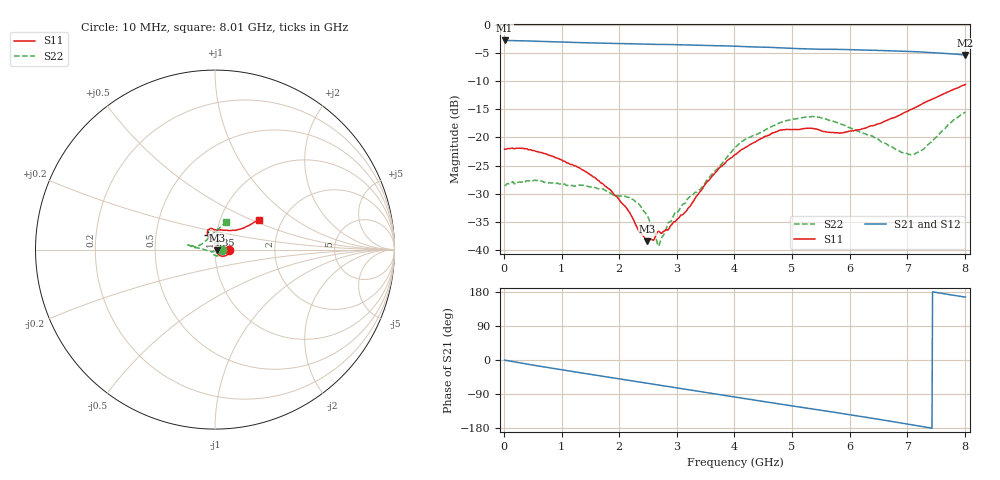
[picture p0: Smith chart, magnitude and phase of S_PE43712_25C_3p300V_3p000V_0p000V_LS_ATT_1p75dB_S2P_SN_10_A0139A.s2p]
! DEVICE ID: PE43712
! File Path: z:\PE43713\PE43713_CHAR_NOM_04292014\AMB\3p300\LS_ATT_1p75dB\PE43713_AMB_3p300V_3p000V_0p000V_LS_ATT_1p75dB_S2P_SN_10_A0139A.s2p
! Serial: 10
! Lot: A0139A
! Temp: 25C
! VDD: 3.300
! VSS: 0.000
! Control_Hi: 3.000
! Control_Lo: 0.000
! Attenuation Step: 1.75dB
! Port 1: RF1
! Port 2: RF2
! ThroughPath:1-2
! IDD: 0.0001468347
! ISS: -9.22e-008
#  Hz  S  RI  R  50
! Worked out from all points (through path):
!   801 points, 10 MHz to 8.01 GHz, reference 50 ohm
!   highest |S21| = -2.79 dB at 10 MHz (marker M1); lowest = -5.4 dB at 8.01 GHz (marker M2)
!   group delay of S21, straight-line fit = 66.5 ps
!   lowest |S11| = -38.4 dB at 2.49 GHz (marker M3), VSWR 1.02, Z = 51.2 - j0.349 ohm
!   |S11| at or under -10 dB: start of sweep to end of sweep
!   |S22| runs from -39.3 to -15.5 dB; largest |S21 - S12| = 0.0022
!   S11 on the Smith chart (normalised r, x): 10 MHz: 1.17, -0.00; 4.35 GHz: 0.91, +0.15; 8.01 GHz: 1.52, +0.55
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1e7  0.0788 -0.000465  0.7254 -0.00398  0.7253 -0.00389  0.0376 -0.000487
6.3e8  0.0679 -0.0283  0.6822 -0.204  0.6818 -0.204  0.0342 -0.0225
1.35e9  0.0364 -0.0369  0.5734 -0.3904  0.5732 -0.3903  0.013 -0.0352
1.84e9  0.0208 -0.0276  0.4764 -0.491  0.4763 -0.4908  0.00131 -0.0322
2.2e9  0.0121 -0.0167  0.3943 -0.5521  0.3944 -0.5518  -0.00773 -0.028
2.35e9  0.0109 -0.00944  0.3574 -0.5733  0.3575 -0.5732  -0.00783 -0.0241
2.49e9  0.0115 -0.00341  0.322 -0.5905  0.3221 -0.5905  -0.00889 -0.018
2.58e9  0.0122 0.00198  0.2991 -0.5996  0.2994 -0.5998  -0.00917 -0.0131
2.68e9  0.0128 0.00724  0.2748 -0.6099  0.275 -0.6098  -0.00668 -0.00853
2.83e9  0.00986 0.0115  0.2352 -0.6254  0.2356 -0.6254  -0.0113 -0.0119
2.97e9  0.00595 0.0169  0.1975 -0.6359  0.1977 -0.6359  -0.0169 -0.0136
3.19e9  -0.000566 0.0233  0.137 -0.6476  0.1371 -0.6477  -0.027 -0.00946
3.72e9  -0.0124 0.051  -0.00763 -0.6513  -0.00755 -0.6512  -0.054 -0.00146
4.01e9  -0.0249 0.0656  -0.0872 -0.6394  -0.0868 -0.6393  -0.081 0.00617
4.35e9  -0.0396 0.0813  -0.1733 -0.6114  -0.173 -0.6115  -0.1041 0.0112
4.8e9  -0.0395 0.1093  -0.279 -0.5584  -0.2784 -0.5586  -0.1344 0.0184
5.35e9  -0.0221 0.1182  -0.3845 -0.4725  -0.3843 -0.472  -0.1511 0.0268
5.86e9  0.0137 0.1085  -0.4692 -0.3801  -0.4682 -0.3802  -0.1291 0.0203
6.68e9  0.0966 0.1069  -0.5547 -0.1919  -0.5545 -0.1916  -0.0803 0.0266
7.02e9  0.1311 0.1114  -0.5701 -0.1058  -0.5695 -0.106  -0.0517 0.0487
7.16e9  0.1468 0.1159  -0.5718 -0.0699  -0.571 -0.0699  -0.0366 0.0631
8.01e9  0.2436 0.1658  -0.5238 0.1299  -0.5223 0.1289  0.0616 0.156
